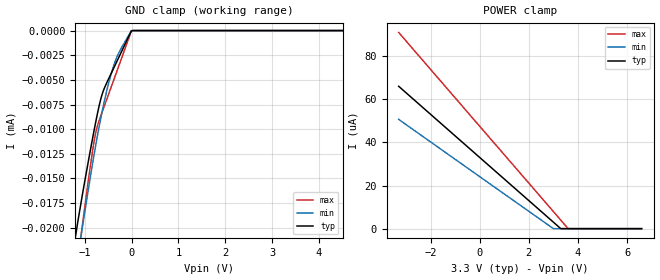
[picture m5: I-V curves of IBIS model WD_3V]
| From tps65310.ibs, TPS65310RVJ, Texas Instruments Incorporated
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[Model]   WD_3V
Model_type   Input
Vinl = .8
Vinh = 2.
|   typ   min   max
C_comp   0.01p   0.01p   0.01p
[Voltage Range]   3.3   3   3.6
[Temperature Range]   27   175   -40
[Power Clamp Reference]   3.3   3   3.6
[GND Clamp Reference]   -0   -0   -0
[GND Clamp]
|   Voltage   I(typ)   I(min)   I(max)
-3.3V     -112.7uA   -95.48uA   -146.7uA
-1.191V   -20.77uA   -24.46uA   -24.97uA
-1.142V   -19.27uA   -22.89uA   -23.14uA
-1.053V   -16.77uA   -20.1uA    -19.88uA
-825mV    -10.78uA   -13.31uA   -12.01uA
-745.8mV  -8.853uA   -11.15uA   -9.993uA
-617.1mV  -6.324uA   -7.99uA    -8.142uA
-508.2mV  -5.089uA   -5.717uA   -6.705uA
-399.3mV  -3.996uA   -3.828uA   -5.268uA
-270.6mV  -2.707uA   -2.247uA   -3.57uA
-3.3mV    -32.11nA   -25.54nA   -42.64nA
6.59V     0A         0A         0A
[POWER Clamp]
|   Voltage   I(typ)   I(min)   I(max)
-3.3V     66.08uA    50.76uA    91.08uA
2.996V    3.038uA    27.94nA    7.963uA
3.293V    64.9nA     0A         4.045uA
3.59V     0A         0A         125.6nA
6.59V     0A         0A         0A
